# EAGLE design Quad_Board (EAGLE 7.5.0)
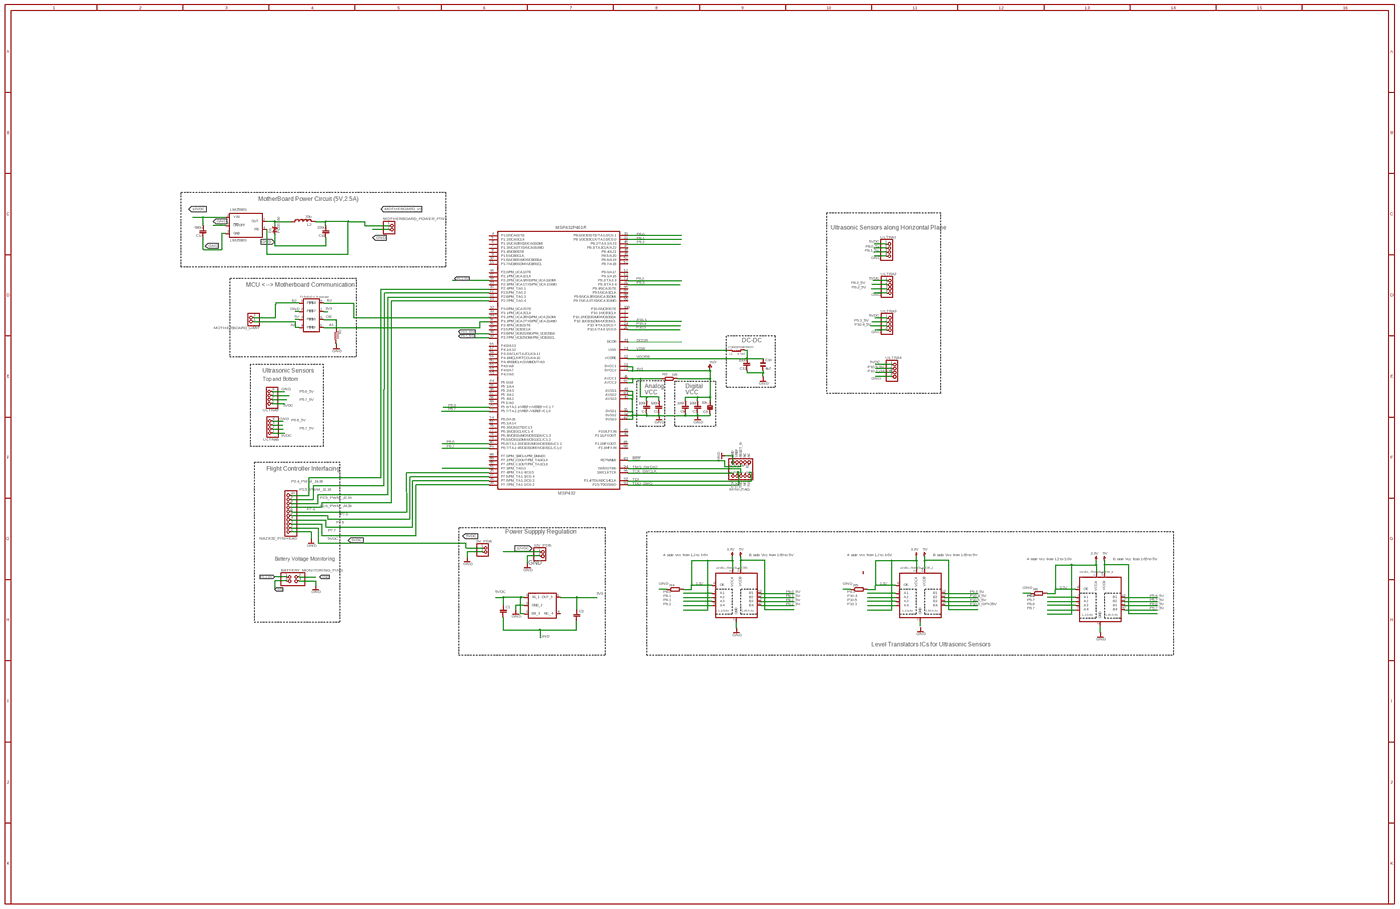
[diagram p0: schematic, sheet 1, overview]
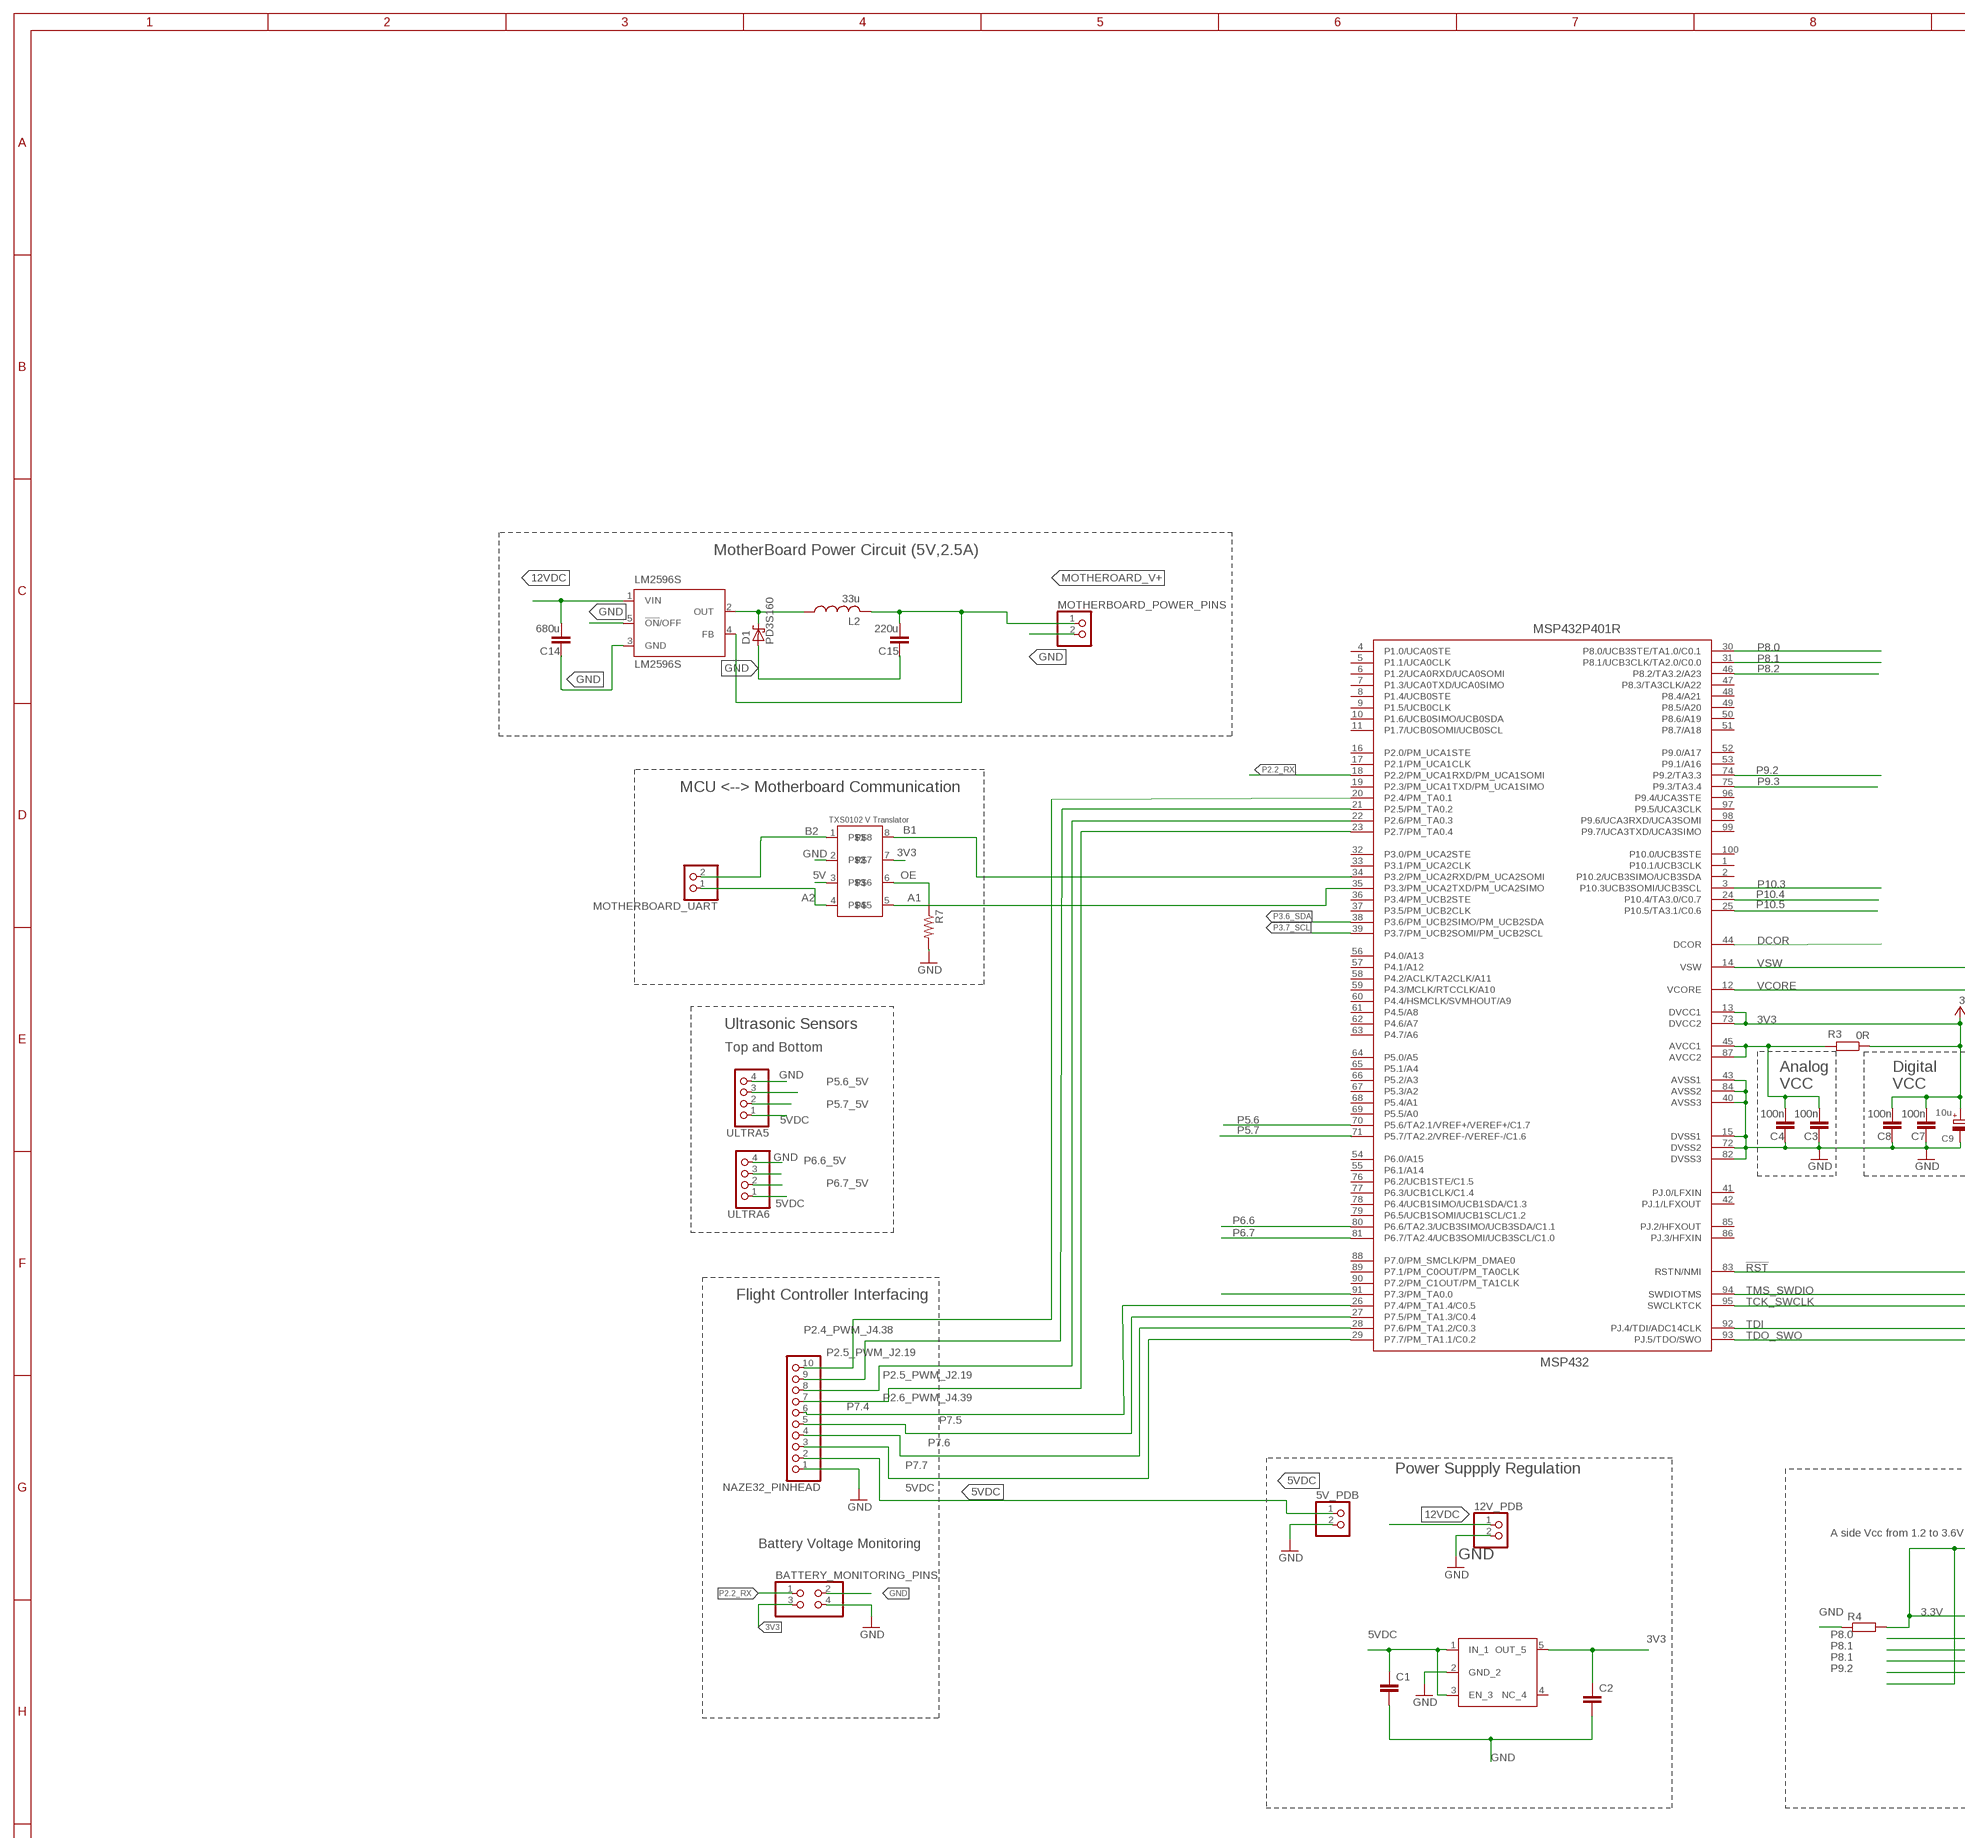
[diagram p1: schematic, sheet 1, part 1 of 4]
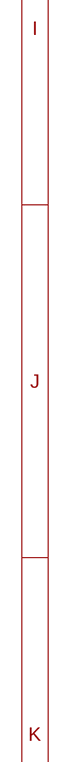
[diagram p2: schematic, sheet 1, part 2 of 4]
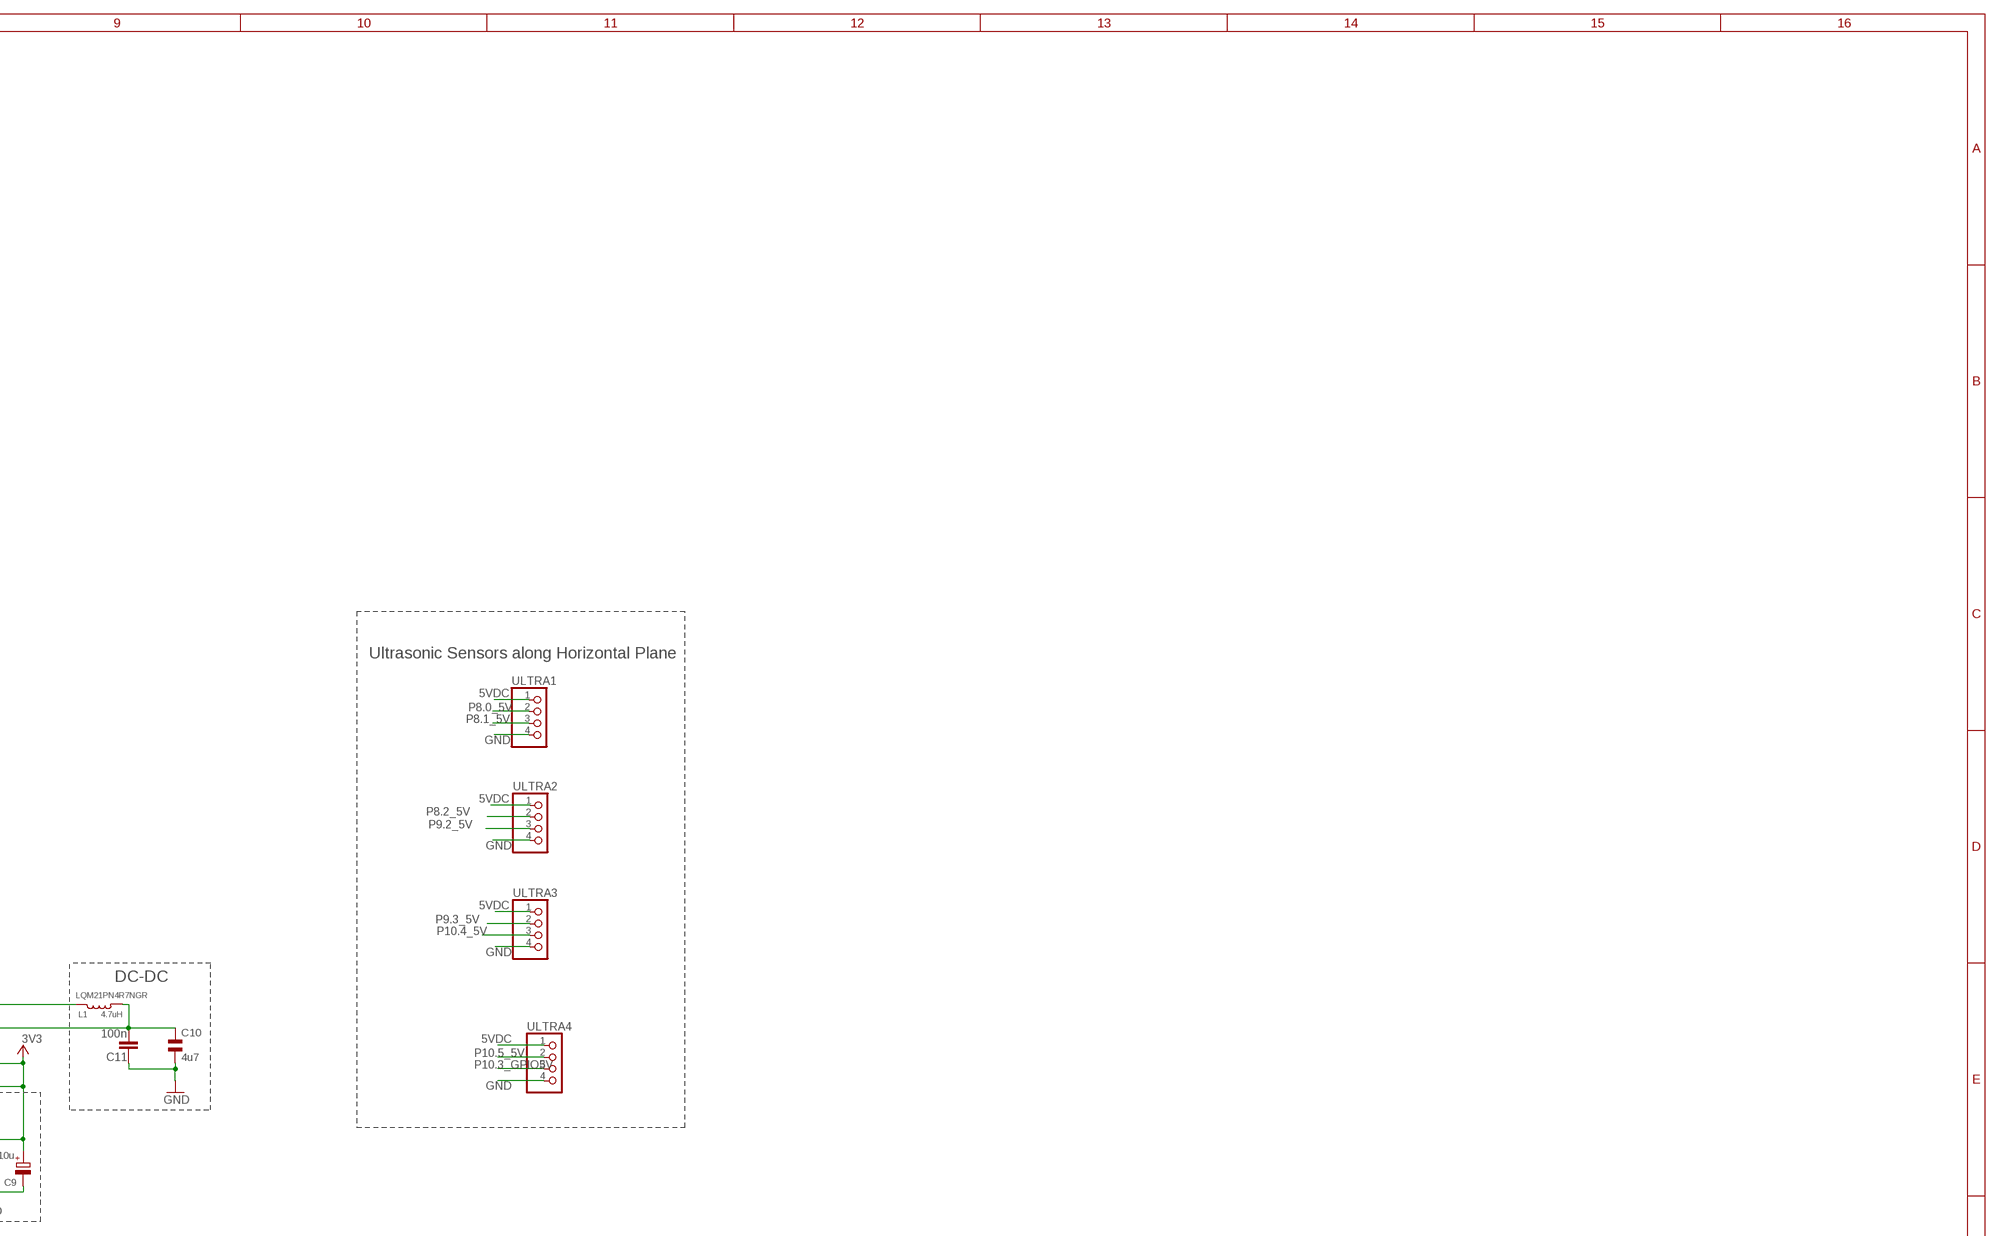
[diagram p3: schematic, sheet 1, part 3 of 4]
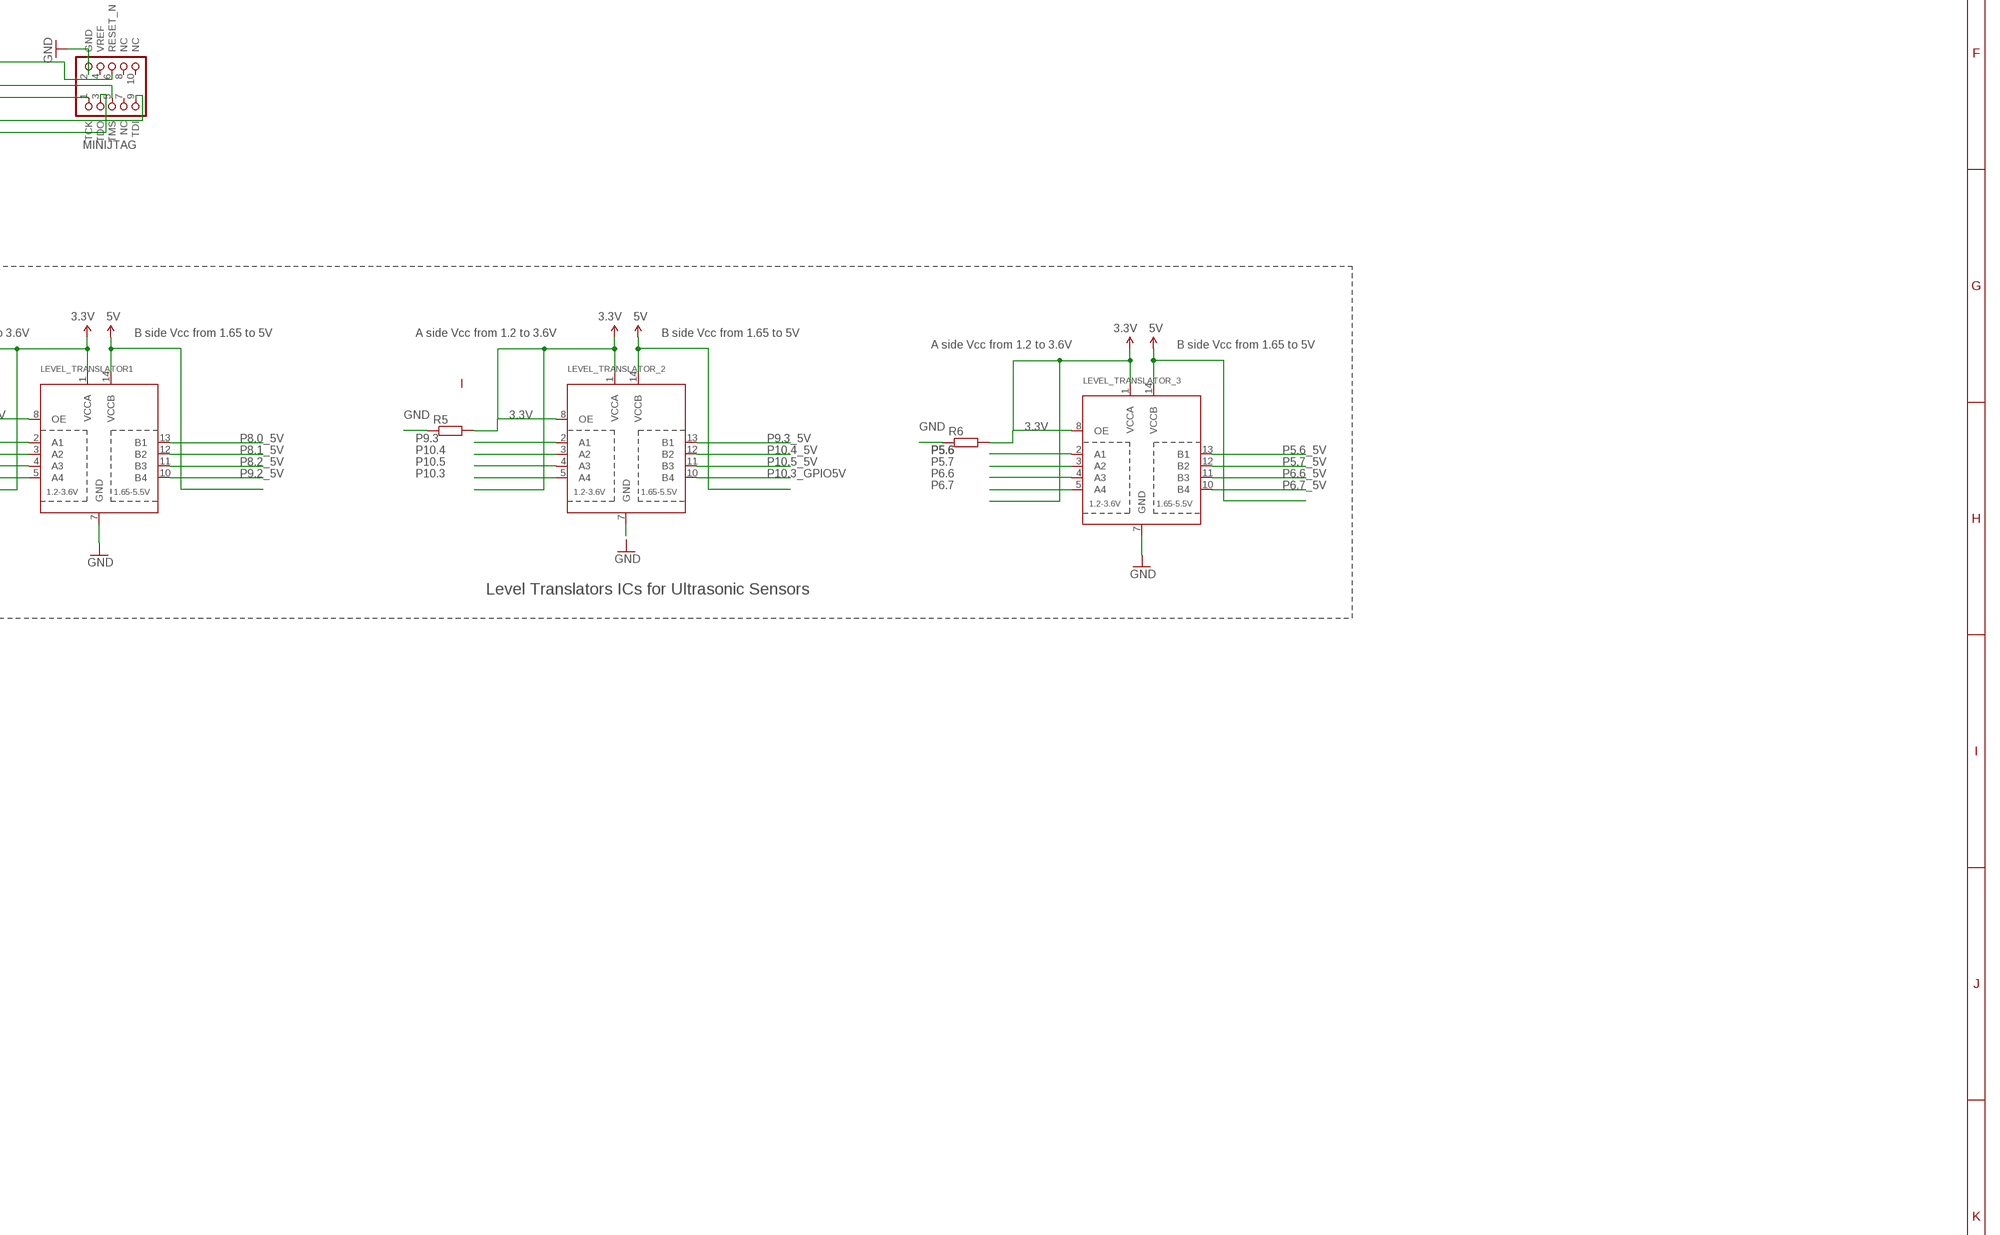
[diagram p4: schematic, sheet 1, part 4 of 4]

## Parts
5V_PDB  PINHD-1X2  [1X02]
12V_PDB  PINHD-1X2  [1X02]
BATTERY_MONITORING_PINS  PINHD-2X2  [2X02]
C1  C2.5/2  [C2.5-2]
C2  C2.5/2  [C2.5-2]
C3  100n  C-EUCM0402  [0402]
C4  100n  C-EUCM0402  [0402]
C7  100n  C-EUCM0402  [0402]
C8  100n  C-EUCM0402  [0402]
C9  10u  CPOL-EUA/3216-18R  [A/3216-18R]
C10  4u7  CSMD0805  [CSMD0805]
C11  100n  C-EUCM0402  [0402]
C14  680u  CC1206  [C1206]
C15  220u  CC1206  [C1206]
D1  PD3S160  [POWERDI323]
L1  4.7uH  LQM2MP_G0  [0806]
L2  33u  L-USL3225M  [L3225M]
LEVEL_TRANSLATOR1  TXB0104PWRSOIC14  [SO14]
LEVEL_TRANSLATOR_2  TXB0104PWRSOIC14  [SO14]
LEVEL_TRANSLATOR_3  TXB0104PWRSOIC14  [SO14]
LM2596S  LM2596S  [TO263-5]
MINIJTAG  JTAG-AVR-IDC  [PAK100/2500-10]
MOTHERBOARD_POWER_PINS  PINHD-1X2  [1X02]
MOTHERBOARD_UART  PINHD-1X2  [1X02]
MSP432P401R  MSP432  [PZ100]
NAZE32_PINHEAD  PINHD-1X10  [1X10]
R3  0R  R-EU_RM0402  [0402]
R4  RR2512  [R2512]
R5  RR2512  [R2512]
R6  RR2512  [R2512]
R7  R-US_0204/5  [0204/5]
U$1  TXS0102  [SM8]
U$2  TLV733P  [SOT23-5]
ULTRA1  PINHD-1X4  [1X04]
ULTRA2  PINHD-1X4  [1X04]
ULTRA3  PINHD-1X4  [1X04]
ULTRA4  PINHD-1X4  [1X04]
ULTRA5  PINHD-1X4  [1X04]
ULTRA6  PINHD-1X4  [1X04]

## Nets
3.3V: LEVEL_TRANSLATOR1.1(VCCA) LEVEL_TRANSLATOR1.8(OE) LEVEL_TRANSLATOR_2.1(VCCA) LEVEL_TRANSLATOR_2.8(OE) LEVEL_TRANSLATOR_3.1(VCCA) LEVEL_TRANSLATOR_3.8(OE) R4.2 R5.2 R6.2
3V3: BATTERY_MONITORING_PINS.3 C2.1 C7.1 C8.1 C9.+ MSP432P401R.13(DVCC1) MSP432P401R.73(DVCC2) R3.1 U$1.7 ; supply symbol labelled +3V3
5V: LEVEL_TRANSLATOR1.14(VCCB) LEVEL_TRANSLATOR_2.14(VCCB) LEVEL_TRANSLATOR_3.14(VCCB) U$1.3
5VDC: 5V_PDB.1 C1.1 NAZE32_PINHEAD.2 U$2.1(IN_1) U$2.3(EN_3) ULTRA1.1 ULTRA2.1 ULTRA3.1 ULTRA4.1 ULTRA5.1 ULTRA6.1
12VDC: 12V_PDB.1 C14.1 LM2596S.1(VIN)
!RST: MINIJTAG.6(RESET_N) MSP432P401R.83(RSTN/NMI)
A1: MSP432P401R.35(P3.3/PM_UCA2TXD/PM_UCA2SIMO) U$1.5
A2: MOTHERBOARD_UART.1 U$1.4
B1: MSP432P401R.34(P3.2/PM_UCA2RXD/PM_UCA2SOMI) U$1.8
B2: MOTHERBOARD_UART.2 U$1.1
DCOR: MSP432P401R.44(DCOR)
GND: 5V_PDB.2 12V_PDB.2 BATTERY_MONITORING_PINS.2 BATTERY_MONITORING_PINS.4 C1.2 C2.2 C3.2 C4.2 C7.2 C8.2 C9.- C10.2 C11.2 C14.2 C15.2 D1.A LEVEL_TRANSLATOR1.7(GND) LEVEL_TRANSLATOR_2.7(GND) LEVEL_TRANSLATOR_3.7(GND) LM2596S.3(GND) LM2596S.5(!ON!/OFF) MINIJTAG.2(GND) MOTHERBOARD_POWER_PINS.2 MSP432P401R.15(DVSS1) MSP432P401R.40(AVSS3) MSP432P401R.43(AVSS1) MSP432P401R.72(DVSS2) MSP432P401R.82(DVSS3) MSP432P401R.84(AVSS2) NAZE32_PINHEAD.1 R4.1 R5.1 R6.1 R7.2 U$1.2 U$2.2(GND_2) ULTRA1.4 ULTRA2.4 ULTRA3.4 ULTRA4.4 ULTRA5.4 ULTRA6.4
MOTHEROARD_V+: C15.1 L2.2 LM2596S.4(FB) MOTHERBOARD_POWER_PINS.1
N$2: C3.1 C4.1 MSP432P401R.45(AVCC1) MSP432P401R.87(AVCC2) R3.2
N$4: D1.C L2.1 LM2596S.2(OUT)
OE: R7.1 U$1.6
P2.2_RX: BATTERY_MONITORING_PINS.1 MSP432P401R.18(P2.2/PM_UCA1RXD/PM_UCA1SOMI)
P2.4_PWM_J4.38: MSP432P401R.20(P2.4/PM_TA0.1) NAZE32_PINHEAD.10
P2.5_PWM_J2.19: MSP432P401R.21(P2.5/PM_TA0.2) NAZE32_PINHEAD.9
P2.6_PWM_J4.39: MSP432P401R.22(P2.6/PM_TA0.3) NAZE32_PINHEAD.8
P2.7_PWM_J4.40: MSP432P401R.23(P2.7/PM_TA0.4) NAZE32_PINHEAD.7
P3.6_SDA: MSP432P401R.38(P3.6/PM_UCB2SIMO/PM_UCB2SDA)
P3.7_SCL: MSP432P401R.39(P3.7/PM_UCB2SOMI/PM_UCB2SCL)
P5.6: LEVEL_TRANSLATOR_3.2(A1) MSP432P401R.70(P5.6/TA2.1/VREF+/VEREF+/C1.7)
P5.6_5V: LEVEL_TRANSLATOR_3.13(B1) ULTRA5.3
P5.7: LEVEL_TRANSLATOR_3.3(A2) MSP432P401R.71(P5.7/TA2.2/VREF-/VEREF-/C1.6)
P5.7_5V: LEVEL_TRANSLATOR_3.12(B2) ULTRA5.2
P6.6: LEVEL_TRANSLATOR_3.4(A3) MSP432P401R.80(P6.6/TA2.3/UCB3SIMO/UCB3SDA/C1.1)
P6.6_5V: LEVEL_TRANSLATOR_3.11(B3) ULTRA6.3
P6.7: LEVEL_TRANSLATOR_3.5(A4) MSP432P401R.81(P6.7/TA2.4/UCB3SOMI/UCB3SCL/C1.0)
P6.7_5V: LEVEL_TRANSLATOR_3.10(B4) ULTRA6.2
P7.3: MSP432P401R.91(P7.3/PM_TA0.0)
P7.4: MSP432P401R.26(P7.4/PM_TA1.4/C0.5) NAZE32_PINHEAD.6
P7.5: MSP432P401R.27(P7.5/PM_TA1.3/C0.4) NAZE32_PINHEAD.5
P7.6: MSP432P401R.28(P7.6/PM_TA1.2/C0.3) NAZE32_PINHEAD.4
P7.7: MSP432P401R.29(P7.7/PM_TA1.1/C0.2) NAZE32_PINHEAD.3
P8.0: LEVEL_TRANSLATOR1.2(A1) MSP432P401R.30(P8.0/UCB3STE/TA1.0/C0.1)
P8.0_5V: LEVEL_TRANSLATOR1.13(B1) ULTRA1.2
P8.1: LEVEL_TRANSLATOR1.3(A2) LEVEL_TRANSLATOR1.4(A3) MSP432P401R.31(P8.1/UCB3CLK/TA2.0/C0.0)
P8.1_5V: LEVEL_TRANSLATOR1.12(B2) ULTRA1.3
P8.2: MSP432P401R.46(P8.2/TA3.2/A23)
P8.2_5V: LEVEL_TRANSLATOR1.11(B3) ULTRA2.2
P9.2: LEVEL_TRANSLATOR1.5(A4) MSP432P401R.74(P9.2/TA3.3)
P9.2_5V: LEVEL_TRANSLATOR1.10(B4) ULTRA2.3
P9.3: LEVEL_TRANSLATOR_2.2(A1) MSP432P401R.75(P9.3/TA3.4)
P9.3_5V: LEVEL_TRANSLATOR_2.13(B1) ULTRA3.2
P10.3: LEVEL_TRANSLATOR_2.5(A4) MSP432P401R.3(P10.3UCB3SOMI/UCB3SCL)
P10.3_GPIO5V: LEVEL_TRANSLATOR_2.10(B4) ULTRA4.3
P10.4: LEVEL_TRANSLATOR_2.3(A2) MSP432P401R.24(P10.4/TA3.0/C0.7)
P10.4_5V: LEVEL_TRANSLATOR_2.12(B2) ULTRA3.3
P10.5: LEVEL_TRANSLATOR_2.4(A3) MSP432P401R.25(P10.5/TA3.1/C0.6)
P10.5_5V: LEVEL_TRANSLATOR_2.11(B3) ULTRA4.2
TCK_SWCLK: MINIJTAG.1(TCK) MSP432P401R.95(SWCLKTCK)
TDI: MINIJTAG.9(TDI) MSP432P401R.92(PJ.4/TDI/ADC14CLK)
TDO_SWO: MINIJTAG.3(TDO) MSP432P401R.93(PJ.5/TDO/SWO)
TMS_SWDIO: MINIJTAG.5(TMS) MSP432P401R.94(SWDIOTMS)
VCORE: C10.1 C11.1 L1.1 MSP432P401R.12(VCORE)
VSW: L1.2 MSP432P401R.14(VSW)
Unconnected: MINIJTAG.4(VREF) MINIJTAG.7(NC) MINIJTAG.8(NC) MINIJTAG.10(NC) U$2.4(NC_4) U$2.5(OUT_5)

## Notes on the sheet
- MotherBoard Power Circuit (5V,2.5A)
- Ultrasonic Sensors along Horizontal Plane
- MCU <--> Motherboard Communication
- DC-DC
- LQM21PN4R7NGR
- Ultrasonic Sensors
- Top and Bottom
- Analog | Digital
- VCC | VCC
- Flight Controller Interfacing
- Power Suppply Regulation
- A side Vcc from 1.2 to 3.6V | B side Vcc from 1.65 to 5V | A side Vcc from 1.2 to 3.6V | B side Vcc from 1.65 to 5V
- Battery Voltage Monitoring | A side Vcc from 1.2 to 3.6V | B side Vcc from 1.65 to 5V
- Level Translators ICs for Ultrasonic Sensors

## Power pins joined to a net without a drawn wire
P1.0/UCA0STE: MSP432P401R.4(P1.0/UCA0STE)
P1.1/UCA0CLK: MSP432P401R.5(P1.1/UCA0CLK)
P1.2/UCA0RXD/UCA0SOMI: MSP432P401R.6(P1.2/UCA0RXD/UCA0SOMI)
P1.3/UCA0TXD/UCA0SIMO: MSP432P401R.7(P1.3/UCA0TXD/UCA0SIMO)
P1.4/UCB0STE: MSP432P401R.8(P1.4/UCB0STE)
P1.5/UCB0CLK: MSP432P401R.9(P1.5/UCB0CLK)
P1.6/UCB0SIMO/UCB0SDA: MSP432P401R.10(P1.6/UCB0SIMO/UCB0SDA)
P1.7/UCB0SOMI/UCB0SCL: MSP432P401R.11(P1.7/UCB0SOMI/UCB0SCL)
P2.0/PM_UCA1STE: MSP432P401R.16(P2.0/PM_UCA1STE)
P2.1/PM_UCA1CLK: MSP432P401R.17(P2.1/PM_UCA1CLK)
P2.3/PM_UCA1TXD/PM_UCA1SIMO: MSP432P401R.19(P2.3/PM_UCA1TXD/PM_UCA1SIMO)
P3.0/PM_UCA2STE: MSP432P401R.32(P3.0/PM_UCA2STE)
P3.1/PM_UCA2CLK: MSP432P401R.33(P3.1/PM_UCA2CLK)
P3.4/PM_UCB2STE: MSP432P401R.36(P3.4/PM_UCB2STE)
P3.5/PM_UCB2CLK: MSP432P401R.37(P3.5/PM_UCB2CLK)
P4.0/A13: MSP432P401R.56(P4.0/A13)
P4.1/A12: MSP432P401R.57(P4.1/A12)
P4.2/ACLK/TA2CLK/A11: MSP432P401R.58(P4.2/ACLK/TA2CLK/A11)
P4.3/MCLK/RTCCLK/A10: MSP432P401R.59(P4.3/MCLK/RTCCLK/A10)
P4.4/HSMCLK/SVMHOUT/A9: MSP432P401R.60(P4.4/HSMCLK/SVMHOUT/A9)
P4.5/A8: MSP432P401R.61(P4.5/A8)
P4.6/A7: MSP432P401R.62(P4.6/A7)
P4.7/A6: MSP432P401R.63(P4.7/A6)
P5.0/A5: MSP432P401R.64(P5.0/A5)
P5.1/A4: MSP432P401R.65(P5.1/A4)
P5.2/A3: MSP432P401R.66(P5.2/A3)
P5.3/A2: MSP432P401R.67(P5.3/A2)
P5.4/A1: MSP432P401R.68(P5.4/A1)
P5.5/A0: MSP432P401R.69(P5.5/A0)
P6.0/A15: MSP432P401R.54(P6.0/A15)
P6.1/A14: MSP432P401R.55(P6.1/A14)
P6.2/UCB1STE/C1.5: MSP432P401R.76(P6.2/UCB1STE/C1.5)
P6.3/UCB1CLK/C1.4: MSP432P401R.77(P6.3/UCB1CLK/C1.4)
P6.4/UCB1SIMO/UCB1SDA/C1.3: MSP432P401R.78(P6.4/UCB1SIMO/UCB1SDA/C1.3)
P6.5/UCB1SOMI/UCB1SCL/C1.2: MSP432P401R.79(P6.5/UCB1SOMI/UCB1SCL/C1.2)
P7.0/PM_SMCLK/PM_DMAE0: MSP432P401R.88(P7.0/PM_SMCLK/PM_DMAE0)
P7.1/PM_C0OUT/PM_TA0CLK: MSP432P401R.89(P7.1/PM_C0OUT/PM_TA0CLK)
P7.2/PM_C1OUT/PM_TA1CLK: MSP432P401R.90(P7.2/PM_C1OUT/PM_TA1CLK)
P8.3/TA3CLK/A22: MSP432P401R.47(P8.3/TA3CLK/A22)
P8.4/A21: MSP432P401R.48(P8.4/A21)
P8.5/A20: MSP432P401R.49(P8.5/A20)
P8.6/A19: MSP432P401R.50(P8.6/A19)
P8.7/A18: MSP432P401R.51(P8.7/A18)
P9.0/A17: MSP432P401R.52(P9.0/A17)
P9.1/A16: MSP432P401R.53(P9.1/A16)
P9.4/UCA3STE: MSP432P401R.96(P9.4/UCA3STE)
P9.5/UCA3CLK: MSP432P401R.97(P9.5/UCA3CLK)
P9.6/UCA3RXD/UCA3SOMI: MSP432P401R.98(P9.6/UCA3RXD/UCA3SOMI)
P9.7/UCA3TXD/UCA3SIMO: MSP432P401R.99(P9.7/UCA3TXD/UCA3SIMO)
P10.0/UCB3STE: MSP432P401R.100(P10.0/UCB3STE)
P10.1/UCB3CLK: MSP432P401R.1(P10.1/UCB3CLK)
P10.2/UCB3SIMO/UCB3SDA: MSP432P401R.2(P10.2/UCB3SIMO/UCB3SDA)
PJ.0/LFXIN: MSP432P401R.41(PJ.0/LFXIN)
PJ.1/LFXOUT: MSP432P401R.42(PJ.1/LFXOUT)
PJ.2/HFXOUT: MSP432P401R.85(PJ.2/HFXOUT)
PJ.3/HFXIN: MSP432P401R.86(PJ.3/HFXIN)

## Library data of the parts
5V_PDB 12V_PDB MOTHERBOARD_POWER_PINS MOTHERBOARD_UART = pinhead:PINHD-1X2: PIN HEADER
BATTERY_MONITORING_PINS = pinhead:PINHD-2X2: PIN HEADER
C1 C2 = capacitor-wima:C: CAPACITOR
C3 C4 C7 C8 C11 = rcl:C-EU: CAPACITOR, European symbol
C9 = rcl:CPOL-EU: POLARIZED CAPACITOR, European symbol
C10 = cap:CSMD0805
C14 C15 = eagle-ltspice:C: CAPACITOR, European symbol; SPICEMODEL: NONE; SPICEPREFIX: C
D1 = diode:PD3S160: 1.0A SURFACE MOUNT SCHOTTKY BARRIER RECTIFIER POWERDI ® 323
L1 = Murata:LQM2MP_G0
L2 = resistor:L-US: INDUCTOR, American symbol
LEVEL_TRANSLATOR1 LEVEL_TRANSLATOR_2 LEVEL_TRANSLATOR_3 = SparkFun-DigitalIC:TXB0104PWR: 4-Bit Bi-Directional Level Shifter 1.2V-3.6V (VCCA) to 1.65V-5.5V (VCCB) bi-directional level shifter with auto direction sensing. Max data rate - VCCA 1.8V: 20Mbps (50ns), VCCA 3.3V: 100Mbps (10ns) Digikey: 296-21929-1-ND (TSSOP) IC-11329; PROD_ID: IC-11329
LM2596S = national-semiconductor:LM2596: SIMPLE SWITCHER® Power Converter 150 kHz 3A Step-Down Voltage Regulator Source: http://www.national.com/ds/LM/LM2596.pdf; MF: NATIONAL SEMICONDUCTOR; MPN: LM2596S-ADJ/NOPB; OC_FARNELL: 9494367; OC_NEWARK: 41K3842
MINIJTAG = kblom:JTAG-AVR: Atmel AVR JTAG source (AVR32) con
MSP432P401R = MSP-EXP432:MSP432
NAZE32_PINHEAD = pinhead:PINHD-1X10: PIN HEADER
R3 = rcl:R-EU_: RESISTOR, European symbol
R4-R6 = eagle-ltspice:R: RESISTOR, European symbol; SPICEMODEL: NONE; SPICEPREFIX: R
R7 = rcl:R-US_: RESISTOR, American symbol
U$1 = TXS0102-bi-directional-translator:TXS0102: Texas Instruments Bi-Driectional Voltage Level Translator Reference - http://www.ti.com/lit/ds/symlink/txs0102.pdf
U$2 = texas:TLV733P: Low Dropout Voltage LDO (Capacitor Free) 300mA 3.3V
ULTRA1-ULTRA6 = pinhead:PINHD-1X4: PIN HEADER

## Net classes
0 default: width 0.254 mm

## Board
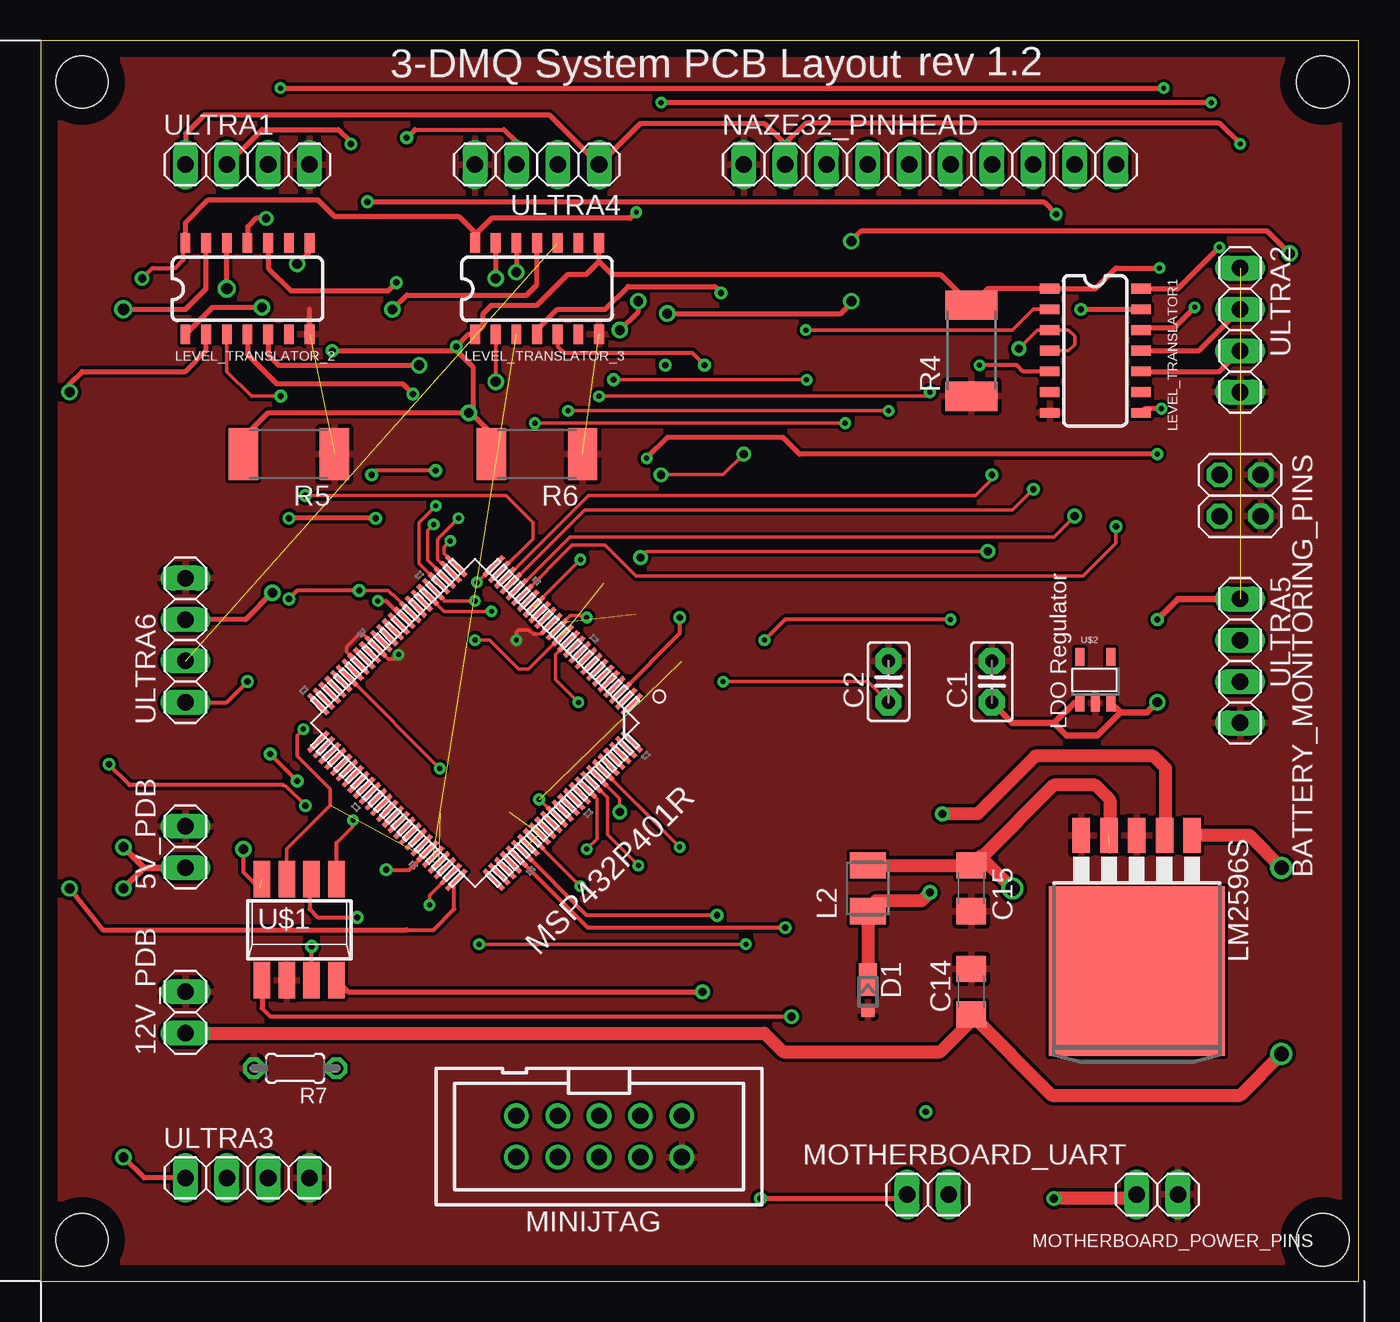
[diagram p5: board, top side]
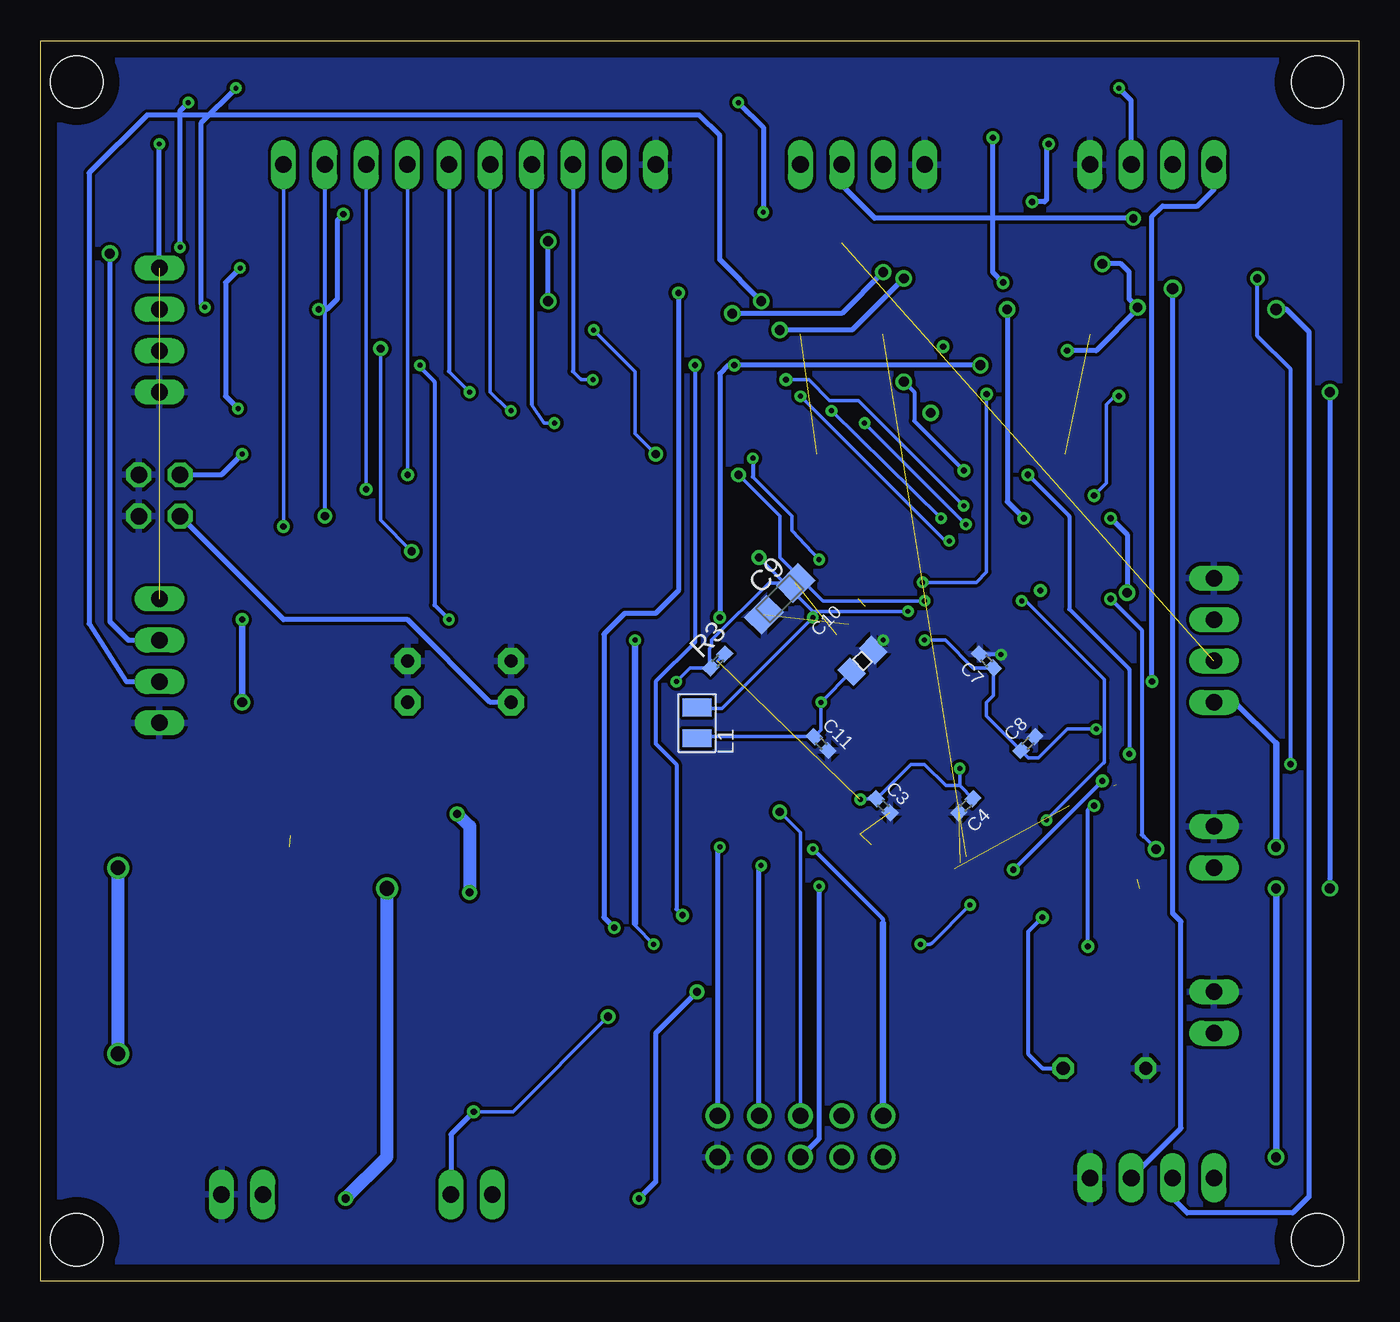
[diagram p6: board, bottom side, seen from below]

Size 80.95 x 76.19 mm. Coordinates in mm from the lower left corner, seen from the top.
Outline: 0,0 80.95,0 80.95,76.19 0,76.19 0,0
Copper layers (1*16): Top 0.035mm / dielectric 1.5mm / Bottom 0.035mm
Design rules "default": minimum track width 10mil, minimum drill 24mil, track to track 8mil, track to pad 8mil, pad to pad 8mil, via to via 8mil, smd to smd 8mil, copper to edge 40mil, drill to drill 8mil, minimum pad ring 10mil, minimum via ring 8mil, stop-mask expansion 4mil, vias tented up to drill 0mil, thermal gap 10mil
Holes 3.2 mm at 2.54,2.54 78.74,2.54 2.54,73.66 78.74,73.66

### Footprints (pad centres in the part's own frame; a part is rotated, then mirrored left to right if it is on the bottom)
1X02 = drill 1.016 long: 1 -1.27,0; 2 1.27,0
2X02 = drill 1.016 octagon: 1 -1.27,-1.27; 2 -1.27,1.27; 3 1.27,-1.27; 4 1.27,1.27
C2.5-2 = drill 0.813 pad 1.6 octagon: 1 -1.27,0; 2 1.27,0
0402 = smd 0.8 x 0.7: 1 -0.6,0; 2 0.6,0
A/3216-18R = smd 1.95 x 1.5: + 1.375,0; - -1.375,0
CSMD0805 = smd 1.092 x 1.397: 1 -0.94,0; 2 0.94,0
C1206 = smd 1.6 x 1.8: 1 -1.4,0; 2 1.4,0
POWERDI323 = smd 0.8 x 0.8: A 1.15,0 | smd 2 x 1.1: C -0.75,0
0806 = smd 1.1 x 1.8: 1 -0.94,0; 2 0.94,0
L3225M = smd 1.6 x 2.2: 1 -1.4,0; 2 1.4,0
SO14 = smd 0.6 x 1.2: 1 -3.81,-2.8; 2 -2.54,-2.8; 3 -1.27,-2.8; 4 0,-2.8; 5 1.27,-2.8; 6 2.54,-2.8; 7 3.81,-2.8; 8 3.81,2.8; 9 2.54,2.8; 10 1.27,2.8; 11 0,2.8; 12 -1.27,2.8; 13 -2.54,2.8; 14 -3.81,2.8
TO263-5 = smd 1.067 x 2.159: 1 -3.404,-5.791; 2 -1.702,-5.791; 3 0,-5.791; 4 1.702,-5.791; 5 3.404,-5.791 | smd 10.8 x 10.41: 6 0,2.54
PAK100/2500-10 = drill 1 pad 1.422: 1 -5.08,-1.27; 2 -5.08,1.27; 3 -2.54,-1.27; 4 -2.54,1.27; 5 0,-1.27; 6 0,1.27; 7 2.54,-1.27; 8 2.54,1.27; 9 5.08,-1.27; 10 5.08,1.27
PZ100 = smd 1.676 x 0.279: 1 -7.62,5.994; 2 -7.62,5.512; 3 -7.62,5.004; 4 -7.62,4.496; 5 -7.62,3.988; 6 -7.62,3.505; 7 -7.62,2.997; 8 -7.62,2.489; 9 -7.62,2.007; 10 -7.62,1.499; 11 -7.62,0.991; 12 -7.62,0.508; 13 -7.62,0; 14 -7.62,-0.508; 15 -7.62,-0.991; 16 -7.62,-1.499; 17 -7.62,-2.007; 18 -7.62,-2.489; 19 -7.62,-2.997; 20 -7.62,-3.505; 21 -7.62,-3.988; 22 -7.62,-4.496; 23 -7.62,-5.004; 24 -7.62,-5.512; 25 -7.62,-5.994; 51 7.62,-5.994; 52 7.62,-5.512; 53 7.62,-5.004; 54 7.62,-4.496; 55 7.62,-3.988; 56 7.62,-3.505; 57 7.62,-2.997; 58 7.62,-2.489; 59 7.62,-2.007; 60 7.62,-1.499; 61 7.62,-0.991; 62 7.62,-0.508; 63 7.62,0; 64 7.62,0.508; 65 7.62,0.991; 66 7.62,1.499; 67 7.62,2.007; 68 7.62,2.489; 69 7.62,2.997; 70 7.62,3.505; 71 7.62,3.988; 72 7.62,4.496; 73 7.62,5.004; 74 7.62,5.512; 75 7.62,5.994 | smd 0.279 x 1.676: 26 -5.994,-7.62; 27 -5.512,-7.62; 28 -5.004,-7.62; 29 -4.496,-7.62; 30 -3.988,-7.62; 31 -3.505,-7.62; 32 -2.997,-7.62; 33 -2.489,-7.62; 34 -2.007,-7.62; 35 -1.499,-7.62; 36 -0.991,-7.62; 37 -0.508,-7.62; 38 0,-7.62; 39 0.508,-7.62; 40 0.991,-7.62; 41 1.499,-7.62; 42 2.007,-7.62; 43 2.489,-7.62; 44 2.997,-7.62; 45 3.505,-7.62; 46 3.988,-7.62; 47 4.496,-7.62; 48 5.004,-7.62; 49 5.512,-7.62; 50 5.994,-7.62; 76 5.994,7.62; 77 5.512,7.62; 78 5.004,7.62; 79 4.496,7.62; 80 3.988,7.62; 81 3.505,7.62; 82 2.997,7.62; 83 2.489,7.62; 84 2.007,7.62; 85 1.499,7.62; 86 0.991,7.62; 87 0.508,7.62; 88 0,7.62; 89 -0.508,7.62; 90 -0.991,7.62; 91 -1.499,7.62; 92 -2.007,7.62; 93 -2.489,7.62; 94 -2.997,7.62; 95 -3.505,7.62; 96 -3.988,7.62; 97 -4.496,7.62; 98 -5.004,7.62; 99 -5.512,7.62; 100 -5.994,7.62
1X10 = drill 1.016 long: 1 -11.43,0; 2 -8.89,0; 3 -6.35,0; 4 -3.81,0; 5 -1.27,0; 6 1.27,0; 7 3.81,0; 8 6.35,0; 9 8.89,0; 10 11.43,0
R2512 = smd 1.8 x 3.2: 1 -2.8,0; 2 2.8,0
0204/5 = drill 0.813 octagon: 1 -2.54,0; 2 2.54,0
SM8 = smd 1.016 x 2.235: 1 -2.286,-3.099; 2 -0.762,-3.099; 3 0.762,-3.099; 4 2.286,-3.099; 5 2.286,3.099; 6 0.762,3.099; 7 -0.762,3.099; 8 -2.286,3.099
SOT23-5 = smd 0.55 x 1.1: 1 -0.95,-1.3; 2 0,-1.3; 3 0.95,-1.3; 4 0.95,1.5; 5 -0.95,1.5
1X04 = drill 1.016 long: 1 -3.81,0; 2 -1.27,0; 3 1.27,0; 4 3.81,0

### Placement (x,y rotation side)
5V_PDB  8.89,26.67 90 top
12V_PDB  8.89,16.51 90 top
BATTERY_MONITORING_PINS  73.66,48.26 270 top
C1  58.42,36.83 90 top
C2  52.07,36.83 90 top
C3  29.21,29.21 315 bottom
C4  24.13,29.21 225 bottom
C7  22.86,38.1 135 bottom
C8  20.32,33.02 45 bottom
C9  35.56,41.91 45 bottom
C10  30.48,38.1 45 bottom
C11  33.02,33.02 315 bottom
C14  57.15,17.78 90 top
C15  57.15,24.13 270 top
D1  50.8,17.78 270 top
L1  40.64,34.29 90 bottom
L2  50.8,24.13 90 top
LEVEL_TRANSLATOR1  64.77,57.15 270 top
LEVEL_TRANSLATOR_2  12.7,60.96 0 top
LEVEL_TRANSLATOR_3  30.48,60.96 0 top
LM2596S  67.31,21.59 180 top
MINIJTAG  34.29,8.89 180 top
MOTHERBOARD_POWER_PINS  68.58,5.33 0 top
MOTHERBOARD_UART  54.48,5.33 0 top
MSP432P401R  26.67,34.29 225 top
NAZE32_PINHEAD  54.61,68.58 0 top
R3  39.37,38.1 45 bottom
R4  57.15,57.15 90 top
R5  15.24,50.8 180 top
R6  30.48,50.8 180 top
R7  15.62,13.08 180 top
U$1  15.88,21.59 0 top
U$2  64.77,36.83 0 top
ULTRA1  12.7,68.58 0 top
ULTRA2  73.66,58.42 270 top
ULTRA3  12.7,6.35 0 top
ULTRA4  30.48,68.58 180 top
ULTRA5  73.66,38.1 270 top
ULTRA6  8.89,39.37 90 top

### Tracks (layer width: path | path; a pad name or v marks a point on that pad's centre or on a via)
3.3V  (via drill 0.3, 0.38, 0.6)
  Top 0.305: LEVEL_TRANSLATOR_2.1 10.55,59.82 v13.59,59.82 | v15.75,62.48 16.51,63.25 LEVEL_TRANSLATOR_2.8 | 27.94,51.06 R6.2 27.69,52.07 26.42,53.34 v26.29,53.34 | 34.29,62.61 LEVEL_TRANSLATOR_3.8 | v68.71,62.23 66.04,62.23 64.77,60.96 LEVEL_TRANSLATOR1.1 58.16,60.96 R4.2 | v68.83,53.59 67.82,53.59 LEVEL_TRANSLATOR1.8 | 56.89,59.95 R4.2 | R5.2 12.44,51.81 13.97,53.34 v26.29,53.34 | v25.53,57.4 26.28,58.16 LEVEL_TRANSLATOR_3.1 27.18,58.67 27.18,59.44 27.69,59.94 30.48,59.94 32.38,61.85 33.53,61.85 34.29,62.61 | v17.91,57.15 25.27,57.15 v25.53,57.4 | R4.2 55.25,61.85 35.05,61.85 34.29,62.61 | v25.53,57.4 25.53,57.15 26.54,56.13 26.54,53.59 v26.29,53.34
  Bottom 0.305: v15.75,62.48 14.61,62.48 14.1,61.98 14.1,60.33 v13.59,59.82 13.59,59.69 16.13,57.15 v17.91,57.15 | v68.71,62.23 69.6,61.34 69.6,54.36 v68.83,53.59
3V3  (via drill 0.3)  (2 unrouted)
  Top 0.203: v26.67,39.37 27.56,39.37 29.34,37.59 29.97,37.59 MSP432P401R.13 | U$1.7 15.11,26.54 17.78,29.21 17.78,30.23 15.75,32.26 15.75,33.53 v16.13,33.91 | v41.91,36.83 50.8,36.83 C2.1
  Bottom 0.203: v26.67,39.37 25.4,39.37 23.71,37.68 C7.1 22.44,35.98 22.86,35.56 22.86,34.71 C8.1 20.28,32.13 19.68,32.13 17.91,33.91 v16.13,33.91 | v41.91,36.83 41.06,37.68 R3.1 39.88,37.76 39.88,38.86 39.75,38.99 39.75,39.37 36.24,42.88 C9.+
  Bottom 0.305: C2.1 53.34,35.56 58.42,40.64 66.04,40.64 BATTERY_MONITORING_PINS.3
5V  (via drill 0.3, 0.38, 0.5)  (1 unrouted)
  Top 0.203: v16.26,29.21 15.05,30.42
  Top 0.254: U$1.3 v16.64,20.57 | 14.9,30.48 5.46,30.48 v4.19,31.75 | v6.22,61.59 6.86,62.23 8.26,62.23 8.76,62.74 8.76,63.63 LEVEL_TRANSLATOR_2.14
  Top 0.305: LEVEL_TRANSLATOR_2.14 8.89,65.02 10.29,66.42 17.02,66.42 18.03,65.41 25.65,65.41 26.67,64.39 | 26.67,64.39 LEVEL_TRANSLATOR_3.14 | LEVEL_TRANSLATOR1.14 69.85,60.96 v72.39,63.5 | v71.88,72.39 v38.1,72.39 | v36.58,65.66 36.2,65.28 27.69,65.28 26.8,64.39 26.67,64.39
  Bottom 0.254: v16.64,20.57 16.64,28.96 16.51,29.08 16.38,29.08 v16.26,29.21 | v4.19,31.75 4.19,56.01 6.22,58.04 v6.22,61.59
  Bottom 0.305: v72.39,63.5 72.39,71.88 v71.88,72.39 | v38.1,72.39 36.58,70.87 v36.58,65.66
5VDC  (via drill 0.3, 0.38, 0.6)  (1 unrouted)
  Top 0.254: ULTRA6.1 11.43,35.56 v12.7,36.83
  Top 0.305: ULTRA3.1 6.35,6.35 v5.08,7.62 | ULTRA1.1 8.89,70.48 10.03,71.63 31.24,71.63 ULTRA4.1 36.83,71.12 44.45,71.12 45.72,69.85 | 45.72,69.85 NAZE32_PINHEAD.2 | v73.66,69.85 72.39,71.12 46.99,71.12 45.72,69.85
  Top 0.406: 5V_PDB.1 6.35,25.4 | 6.35,25.4 v5.08,26.67 | v5.08,24.13 6.35,25.4 | C1.1 59.69,34.29 62.23,34.29 | 62.23,34.29 63.47,35.53 U$2.1 | ULTRA5.1 69.85,41.91 v68.58,40.64 | v68.58,35.56 67.94,34.92 66.33,34.92 U$2.3 66.29,34.96 66.29,34.92 64.9,33.53 62.99,33.53 62.23,34.29
  Bottom 0.305: 5.08,33.02 7.62,35.56 ULTRA6.1 | v12.7,36.83 12.7,65.41 12.06,66.04 9.91,66.04 8.89,67.06 ULTRA1.1 | ULTRA2.1 v73.66,69.85
  Bottom 0.406: v5.08,26.67 5.08,33.02 | v5.08,7.62 v5.08,24.13 | v68.58,40.64 v68.58,35.56
12VDC  (via drill 0.9)
  Top 0.813: 12V_PDB.1 44.45,15.24 45.59,14.1 55.24,14.1 57.15,16 C14.1 62.1,11.43 73.66,11.43 v76.2,13.97 | v76.2,25.4 74.22,27.38 LM2596S.1
  Bottom 0.813: v76.2,13.97 v76.2,25.4
!RST  (via drill 0.3)
  Top 0.203: MSP432P401R.83 arc45 30.32,27.08 v33.15,24.26
  Bottom 0.305: MINIJTAG.6 33.15,8.76 v33.15,24.26
A1  (via drill 0.3)
  Top 0.203: 18.16,26.92 19.12,27.88 arc45 19.18,28.02 v19.18,28.32
  Top 0.254: U$1.5 18.16,26.92 | v20.7,41.78 21.21,41.78 22.25,40.74 MSP432P401R.35
  Bottom 0.203: v19.18,28.32 15.68,31.82 arc-45 15.62,31.96 15.62,36.96 20.39,41.72 arc-45 20.53,41.78 v20.7,41.78
A2  (via drill 0.38, 0.5)
  Top 0.305: v44.2,5.08 52.96,5.08 MOTHERBOARD_UART.1 | U$1.4 18.87,17.78 v40.64,17.78
  Bottom 0.305: v44.2,5.08 43.18,6.1 43.18,15.24 v40.64,17.78
B1  (via drill 0.38, 0.6)  (1 unrouted)
  Top 0.203: MSP432P401R.34 21.63,42.16 21.59,42.16 21.34,42.42 v19.56,42.42
  Top 0.254: v12.45,26.54 12.45,25.15 13.46,24.13 | v19.56,42.42 15.75,42.42 v15.24,41.91
  Bottom 0.203: 13.21,27.3 v12.45,26.54
  Bottom 0.254: v15.24,41.91 13.34,40.01 13.34,27.43 13.21,27.3
B2  (via drill 0.38, 0.5)
  Top 0.254: 13.59,16.76 14.1,16.26 v46.1,16.26
  Top 0.305: U$1.1 13.59,16.76
  Bottom 0.203: v46.1,16.26 51.94,10.41 v54.36,10.41
  Bottom 0.305: v54.36,10.41 55.75,9.02 MOTHERBOARD_UART.2
GND  (via drill 0.3)  (6 unrouted)
  Top 0.203: v21.97,38.48 21.72,38.23 21.33,38.23 MSP432P401R.40 19.81,39.75 19.56,39.75 18.8,38.99 18.8,38.64 MSP432P401R.43 | v29.21,39.37 29.21,39.88 29.34,40.01 29.97,40.01 30.23,39.75 30.73,39.75 MSP432P401R.15
  Top 0.305: LEVEL_TRANSLATOR_2.7 16.51,59.69
  Bottom 0.203: C10.2 v29.21,39.37
  Bottom 0.254: C7.2 22.01,38.52 v21.97,38.48
  pour Bottom: 0,76.2 0,0 81.28,0 81.28,76.2
  pour Top: 0,76.2 0,0 81.28,0 81.28,76.2
MOTHEROARD_V+  (via drill 0.5, 0.9)  (1 unrouted)
  Top 0.813: L2.2 C15.1 57.72,26.1 | 65.66,26.67 65.66,29.59 64.77,30.48 62.23,30.48 57.85,26.1 57.72,26.1 | MOTHERBOARD_POWER_PINS.1 67.06,5.08 v62.23,5.08 | v59.69,24.13 57.72,26.1
  Bottom 0.813: v62.23,5.08 59.69,7.62 v59.69,24.13
N$2  (via drill 0.3)  (1 unrouted)
  Top 0.203: MSP432P401R.45 18.8,37.08 18.93,37.08 v24.51,31.5 | v30.61,29.59 30.65,29.59 MSP432P401R.87
  Bottom 0.203: v24.51,31.5 24.51,30.44 | 24.51,30.44 C4.1 | 24.51,30.44 25.36,30.44 26.67,31.75 27.52,31.75 C3.1 30.56,29.63 v30.61,29.59 | R3.2 39.37,38.1
N$4  (via drill 0.5)
  Top 0.813: D1.C L2.1 50.8,22.86 51.31,23.37 54.1,23.37 v54.61,23.88 | LM2596S.2 69.09,27.46 69.09,31.5 68.33,32.26 61.09,32.26 57.53,28.7 v55.37,28.7
  Bottom 0.813: v55.37,28.7 54.61,27.94 v54.61,23.88
OE  (via drill 0.38)
  Top 0.254: U$1.6 16.51,24.56 16.51,22.86 17.02,22.35 v19.43,22.35
  Bottom 0.254: v19.43,22.35 20.32,21.46 20.32,13.97 19.43,13.08 R7.1
P2.2_RX  (via drill 0.3)  (1 unrouted)
  Top 0.203: v33.15,44.32 30.73,41.91
  Top 0.305: v68.58,50.8 46.61,50.8 45.59,51.82 38.48,51.82 v37.21,50.55
  Bottom 0.203: 37.21,49.4 34.8,46.99 34.8,46.1 v33.15,44.32
  Bottom 0.254: v37.21,50.55 37.21,49.4
  Bottom 0.305: BATTERY_MONITORING_PINS.1 69.85,49.53 v68.58,50.8
P2.4_PWM_J4.38  (via drill 0.38)
  Top 0.203: MSP432P401R.20 32.64,45.21 34.67,45.21 36.58,43.31 64.01,43.31 66.04,45.34 v66.04,46.35
  Bottom 0.203: v66.04,46.35 NAZE32_PINHEAD.10
P2.5_PWM_J2.19  (via drill 0.5)
  Top 0.203: MSP432P401R.21 29.29,42.5 32.51,45.72 62.23,45.72 v63.5,46.99
  Bottom 0.254: NAZE32_PINHEAD.9 v63.5,46.99
P2.6_PWM_J4.39  (via drill 0.38)
  Top 0.203: MSP432P401R.22 33.4,47.37 59.69,47.37 v60.96,48.64
  Bottom 0.203: v60.96,48.64 NAZE32_PINHEAD.8
P2.7_PWM_J4.40  (via drill 0.38)
  Top 0.203: MSP432P401R.23 28.61,43.22 33.66,48.26 57.4,48.26 58.42,49.28 v58.42,49.53
  Bottom 0.203: v58.42,49.53 NAZE32_PINHEAD.7
P5.6  (via drill 0.38, 0.6)
  Top 0.254: LEVEL_TRANSLATOR_3.2 v27.94,55.24 | v24.26,49.78 20.57,49.78 v20.32,49.53 | v14.1,32.38 v15.75,30.73 | v21.21,25.27 22.61,25.27 MSP432P401R.70
  Bottom 0.254: v27.94,55.24 27.3,54.61 27.3,52.83 v24.26,49.78 | v20.32,49.53 17.78,46.99 17.78,41.27 14.1,37.59 v14.1,32.38 | v15.75,30.73 v21.21,25.27
P5.6_5V  (via drill 0.6)
  Top 0.305: LEVEL_TRANSLATOR_3.13 v27.94,61.59 | v35.56,58.42 36.7,59.56 v36.7,60.2
  Bottom 0.305: v27.94,61.59 31.11,58.42 v35.56,58.42 | v36.7,60.2 39.24,62.74 39.24,70.36 40.51,71.63 74.42,71.63 77.98,68.07 77.98,40.39 75.69,36.83 ULTRA5.3
P5.7  (1 unrouted)
P5.7_5V  (via drill 0.6)
  Top 0.305: LEVEL_TRANSLATOR_3.12 v29.21,61.98 | v38.48,59.44 49.15,59.44 49.78,60.07 v49.78,60.2 | v49.78,63.88 50.42,64.52 75.31,64.52 v76.71,63.12
  Bottom 0.305: v29.21,61.98 31.75,59.44 v38.48,59.44 | v49.78,60.2 v49.78,63.88 | v76.71,63.12 76.71,40.51 75.56,39.37 ULTRA5.2
P6.6  (via drill 0.38)
  Top 0.254: LEVEL_TRANSLATOR_3.4 30.48,58.29 | v45.72,21.72 33.6,21.72 MSP432P401R.80
  Top 0.305: 30.48,58.29 30.48,58.42 31.75,59.69 34.67,59.69 36.07,61.09 41.4,61.09 v41.78,60.71
  Bottom 0.305: v41.78,60.71 41.78,42.42 43.18,41.02 45.09,41.02 46.35,39.75 46.35,22.35 v45.72,21.72
P6.6_5V  (via drill 0.38, 0.6)
  Top 0.305: 30.48,62.99 LEVEL_TRANSLATOR_3.11 30.48,61.21 29.84,60.58 22.48,60.58 v21.59,59.69 | v20.57,46.86 v15.24,46.86 | v14.22,42.29 12.57,40.64 ULTRA6.3
  Bottom 0.305: v21.59,59.69 21.59,47.88 v20.57,46.86 | v15.24,46.86 14.22,45.85 v14.22,42.29
P6.7  (via drill 0.38)
  Top 0.254: LEVEL_TRANSLATOR_3.5 31.75,57.4 32.13,57.02 40.01,57.02 v40.77,56.26 | v41.53,22.48 33.52,22.48 MSP432P401R.81
  Bottom 0.254: v40.77,56.26 40.77,39.24 43.18,36.83 43.18,33.02 41.91,31.75 41.91,22.86 v41.53,22.48
P6.7_5V  (1 unrouted)
P7.4  (via drill 0.3)
  Top 0.203: MSP432P401R.26 arc45 25.5,43.97 24.77,44.7 24.77,45.09 v25.15,45.47 | v34.29,54.36 54.27,54.36 arc45 54.42,54.42 v54.61,54.61
  Bottom 0.203: v25.15,45.47 25.32,45.47 arc45 25.46,45.53 v34.29,54.36 | v54.61,54.61 55.88,55.88
  Bottom 0.254: NAZE32_PINHEAD.6 55.88,55.88
P7.5  (via drill 0.3)
  Top 0.203: MSP432P401R.27 arc-45 25.1,43.61 24.38,44.32 24.38,45.51 arc-45 24.44,45.65 v25.65,46.86 | v32.38,53.47 v52.07,53.47
  Bottom 0.203: NAZE32_PINHEAD.5 53.34,54.61 52.26,53.53 arc-45 52.11,53.47 v52.07,53.47 | v25.65,46.86 v32.38,53.47
P7.6  (via drill 0.3)
  Top 0.203: MSP432P401R.28 23.75,44.29 23.75,46.1 v24.13,46.48 | v30.35,52.7 v49.4,52.7
  Bottom 0.203: v24.13,46.48 v30.35,52.7 | v49.4,52.7 50.04,52.7 50.8,53.85
  Bottom 0.254: NAZE32_PINHEAD.4 50.8,53.85
P7.7  (via drill 0.3, 0.38)
  Top 0.203: MSP432P401R.29 23.24,44.08 23.24,46.61 v24.26,47.62 | v35.18,55.37 v47.03,55.37
  Bottom 0.203: v24.26,47.62 30.73,54.1 32.51,54.1 33.78,55.37 v35.18,55.37 | v47.03,55.37 47.67,55.37 arc45 47.81,55.43 48.26,55.88
  Bottom 0.254: NAZE32_PINHEAD.3 48.26,55.88
P8.0  (via drill 0.3, 0.5)
  Top 0.203: 24.1,42.45 MSP432P401R.30 24.77,41.84 24.77,41.78 v26.67,41.78 | v46.99,58.42 59.69,58.42 60.96,59.69 LEVEL_TRANSLATOR1.2 | v43.18,50.8 41.91,49.53 v38.1,49.53
  Bottom 0.203: v26.67,41.78 32.89,41.78 35.56,44.45 35.56,46.99 v38.1,49.53 | v46.99,58.42 44.45,55.88 44.45,52.07 v43.18,50.8
P8.0_5V  (via drill 0.38)
  Top 0.305: ULTRA1.2 13.59,70.74 18.29,70.74 19.05,69.98 v19.05,69.85 | v20.07,66.29 61.59,66.29 v62.36,65.53 | v63.88,59.69 LEVEL_TRANSLATOR1.13
  Bottom 0.305: v19.05,69.85 19.18,69.72 19.18,66.42 19.3,66.29 v20.07,66.29 | v62.36,65.53 62.74,65.15 62.74,60.33 63.37,59.69 v63.88,59.69
P8.1  (via drill 0.3, 0.5)
  Top 0.203: MSP432P401R.31 24.77,41.15 v27.69,41.15 | v36.83,44.45 37.21,44.83 v58.17,44.83 | v60.07,57.28 61.21,58.42 LEVEL_TRANSLATOR1.3 63.12,58.42 63.5,58.04 63.5,57.53 63.12,57.15 LEVEL_TRANSLATOR1.4
  Bottom 0.203: v27.69,41.15 33.53,41.15 v36.83,44.45 | v58.17,44.83 60.07,46.74 v60.07,57.28
P8.1_5V  (via drill 0.3)
  Top 0.305: v14.73,73.28 v68.96,73.28 | v70.87,59.82 69.6,58.55 67.7,58.55 LEVEL_TRANSLATOR1.12
  Bottom 0.305: ULTRA1.3 13.97,72.52 v14.73,73.28 | v68.96,73.28 71.12,71.12 71.12,60.07 v70.87,59.82
P8.2_5V
  Top 0.305: LEVEL_TRANSLATOR1.11 71.12,57.15 ULTRA2.2
P9.2  (via drill 0.3)
  Top 0.203: MSP432P401R.74 23.94,23.76 arc45 23.88,23.62 v23.88,23.11 | v26.92,20.7 v43.31,20.7
  Top 0.254: LEVEL_TRANSLATOR1.5 60.33,55.88 59.94,56.26 v57.66,56.26 | v55.88,40.64 45.72,40.64 v44.45,39.37
  Bottom 0.203: v23.88,23.11 26.23,20.76 arc45 26.37,20.7 v26.92,20.7 | v43.31,20.7 44.39,21.78 arc45 44.45,21.93 44.45,21.97
  Bottom 0.254: v57.66,56.26 57.66,56.13 56.77,55.24 56.77,41.53 v55.88,40.64
  Bottom 0.406: v44.45,39.37 44.45,21.97
P9.2_5V
  Top 0.305: LEVEL_TRANSLATOR1.10 72.39,55.88 ULTRA2.3
P9.3  (via drill 0.6)
  Top 0.203: 25.52,24.63 MSP432P401R.75
  Top 0.254: 22.48,21.59 24.13,21.59 25.4,22.86 25.4,24.54
  Top 0.305: v1.78,24.13 3.81,21.59 22.48,21.59 | v1.78,54.61 1.78,55.12 2.54,55.88 8.89,55.88 10.16,57.15 LEVEL_TRANSLATOR_2.2 | 25.4,24.54 MSP432P401R.75
  Bottom 0.305: v1.78,54.61 v1.78,24.13
P9.3_5V  (via drill 0.7)
  Top 0.305: v5.08,59.69 8.89,59.69 10.16,60.96 LEVEL_TRANSLATOR_2.13
  Bottom 0.305: v5.08,59.69 4.45,59.69 3.05,58.29 3.05,5.21 4.06,4.19 10.54,4.19 11.43,5.08 ULTRA3.2
P10.3  (via drill 0.38, 0.6)
  Top 0.254: v39.24,40.77 39.24,39.79 MSP432P401R.3
  Top 0.305: LEVEL_TRANSLATOR_2.5 13.97,56.9 14.61,56.26 v23.24,56.26
  Bottom 0.305: v39.24,40.77 39.24,55.75 38.73,56.26 v38.35,56.26 v23.24,56.26
P10.3_GPIO5V  (via drill 0.38)
  Top 0.254: 22.99,70.74 28.45,70.74
  Top 0.305: LEVEL_TRANSLATOR_2.10 13.97,62.23 15.37,60.83 21.34,60.83 v21.84,61.34 | v22.48,70.23 22.99,70.74 | 28.45,70.74 29.21,69.98 ULTRA4.3
  Bottom 0.305: v21.84,61.34 22.48,61.98 v22.48,70.23
P10.4  (via drill 0.38)
  Top 0.203: MSP432P401R.24 28.21,43.58 30.23,45.59 30.23,46.61 28.57,48.26 v16.26,48.26 | LEVEL_TRANSLATOR_2.3 11.43,55.88 12.95,54.36 v14.73,54.36
  Bottom 0.203: v14.73,54.36 14.99,54.36 15.49,53.85 15.49,49.02 v16.26,48.26
P10.4_5V  (via drill 0.7)
  Top 0.305: v11.43,60.96 LEVEL_TRANSLATOR_2.12
  Bottom 0.305: ULTRA3.3 10.92,9.4 10.92,22.1 11.43,22.61 v11.43,60.96
P10.5  (via drill 0.3, 0.38)
  Top 0.203: MSP432P401R.25 27.79,43.92 v26.8,42.93
  Top 0.305: LEVEL_TRANSLATOR_2.4 12.7,56.9 14.48,55.12 22.23,55.12 v22.86,54.48
  Bottom 0.203: v26.8,42.93 23.5,42.93 22.86,43.56 v22.86,54.48
P10.5_5V  (via drill 0.5)
  Top 0.305: v13.84,65.28 13.21,65.28 12.7,64.77 LEVEL_TRANSLATOR_2.11
  Bottom 0.305: ULTRA4.2 31.75,67.31 29.72,65.28 v13.84,65.28
TCK_SWCLK  (via drill 0.3)  (1 unrouted)
  Top 0.203: MSP432P401R.95 v39.24,26.67 36.7,29.21
  Bottom 0.203: v39.24,26.67 39.37,26.54
  Bottom 0.305: 39.37,26.54 MINIJTAG.1
TDI  (via drill 0.3)
  Top 0.203: MSP432P401R.92 34.16,29.64 34.16,27.18 v33.53,26.54
  Bottom 0.254: v33.53,26.54 29.27,22.29 arc45 29.21,22.14 29.21,21.97
  Bottom 0.406: MINIJTAG.9 29.21,21.97
TDO_SWO  (via drill 0.3)
  Top 0.203: MSP432P401R.93 33.85,30.66 34.8,29.72 34.8,27.43 v36.7,25.53
  Bottom 0.305: MINIJTAG.3 36.83,25.32 arc45 36.77,25.46 v36.7,25.53
TMS_SWDIO  (via drill 0.5)
  Top 0.203: v35.56,28.83 35.56,29.64 MSP432P401R.94
  Bottom 0.203: MINIJTAG.5 34.29,27.56 v35.56,28.83
VCORE  (via drill 0.3)
  Top 0.203: MSP432P401R.12 32.42,39.27 31.62,38.48 31.62,36.96 v33.02,35.56
  Bottom 0.203: C10.1 v33.02,35.56 33.02,33.87 C11.1 40.55,33.44 L1.1
VSW  (via drill 0.3)
  Top 0.203: MSP432P401R.14 31.7,40.08 32.51,40.89 33.4,40.89 v33.53,40.77
  Bottom 0.203: v33.53,40.77 39.12,35.18 40.59,35.18 L1.2

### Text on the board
tPlace: 3-DMQ System PCB Layout | rev 1.2
tNames: LDO Regulator

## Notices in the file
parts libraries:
SparkFun-DigitalIC: Licensing: CC v3.0 Share-Alike You are welcome to use this library for commercial purposes.
